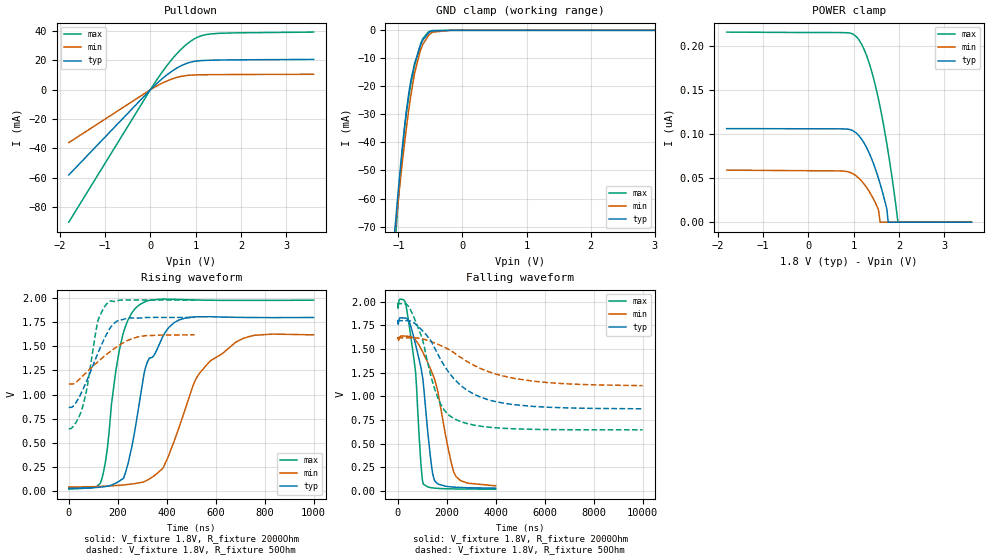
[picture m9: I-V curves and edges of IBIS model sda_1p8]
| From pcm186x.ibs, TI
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|   sda_1p8 Model
[Model]   sda_1p8
Model_type   I/O_open_drain
Polarity   Non-Inverting
Vinl = 0.54
Vinh = 1.26
Vmeas = 0.9
Vref = 1.8
Cref = 400pF
Rref = 2000
|   typ   min   max
|   (nom PVT)   (fast PVT)   (slow PVT)
C_comp   9.904e-12   9.661e-12   1.003e-11
[Model spec]
|subparameter
Vinl   0.54   0.486   0.594
Vinh   1.26   1.134   1.386
| Where nom  PVT is Nominal Process, 1.8V, 27C
|   Fast PVT is Strong Process,  1.98V, -40C
|   Slow PVT is Weak Process,   1.62V, 125C
[Voltage Range]   1.8   1.62   1.98
|Junction Temperature
[Temperature Range]   27   125   -40
[Pullup Reference]   1.8   1.62   1.98
[Pulldown Reference]   0   0   0
[Power Clamp Reference]   1.8   1.62   1.98
[GND Clamp Reference]   0   0   0
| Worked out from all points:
|   slope of the pulldown table from 0 to 0.27 V, typ, clamps not added: 34.7 ohm
|   GND clamp passes 1 mA (typ) near -0.53 V on its own axis
|   falling waveform, V_fixture 1.8V, R_fixture 2000Ohm: 20-80 % time 502ns typ, 817ns min, 358ns max; typ from 1.8 V to 0.031 V
|   rising waveform, V_fixture 1.8V, R_fixture 2000Ohm: 20-80 % time 105ns typ, 156ns min, 61.8ns max; typ from 0.028 V to 1.8 V
|   falling waveform, V_fixture 1.8V, R_fixture 50Ohm: 20-80 % time 1.62us typ, 2.39us min, 912ns max; typ from 1.8 V to 0.87 V
|   rising waveform, V_fixture 1.8V, R_fixture 50Ohm: 20-80 % time 94.1ns typ, 145ns min, 53.8ns max; typ from 0.868 V to 1.8 V
[Pulldown]
|   Voltage   I(typ)   I(min)   I(max)
-1.8V     -58.2mA    -36.13mA   -90.43mA
130.5mV   3.944mA    2.382mA    6.262mA
277mV     7.97mA     4.736mA    12.81mA
482.6mV   12.8mA     7.39mA     21.04mA
644.4mV   15.83mA    8.868mA    26.59mA
821.2mV   18.2mA     9.793mA    31.57mA
1.054V    19.71mA    10.17mA    36.04mA
1.331V    20.16mA    10.29mA    38.09mA
1.978V    20.42mA    10.4mA     38.88mA
3.6V      20.7mA     10.55mA    39.35mA
[GND Clamp]
|   Voltage   I(typ)   I(min)   I(max)
-1.8V     -364.4mA   -298.1mA   -450.1mA
-1.051V   -70.48mA   -71.85mA   -76.76mA
-1.003V   -57.72mA   -61.01mA   -61.48mA
-964.4mV  -48.15mA   -52.71mA   -50.3mA
-903.1mV  -34.39mA   -40.29mA   -35.2mA
-875mV    -28.89mA   -35mA      -29.71mA
-806.4mV  -18.17mA   -23.43mA   -19.44mA
-747mV    -11.85mA   -15.4mA    -12.68mA
-655.6mV  -5.372mA   -7.194mA   -5.046mA
-522.9mV  -763.3uA   -1.643mA   -392.6uA
-180mV    -66.44nA   -963.5nA   -79.79nA
3.6V      0A         0A         0A
[POWER Clamp]
|   Voltage   I(typ)   I(min)   I(max)
-1.8V     106.1nA    59.03nA    215.6nA
748.3mV   105.8nA    58.08nA    215nA
1.01V     102.9nA    54.12nA    212.5nA
1.237V    89.12nA    42.81nA    195.1nA
1.385V    73.37nA    31.25nA    173.3nA
1.485V    59.61nA    21.38nA    153.8nA
1.55V     49.37nA    13.69nA    139nA
1.584V    43.58nA    0A         130.7nA
1.732V    14.91nA    0A         88.82nA
1.762V    0A         0A         79.37nA
1.978V    0A         0A         0A
3.6V      0A         0A         0A
[Ramp]
R_load = 2000
|   typ   min   max
dV/dt_r   1.0624/1.05238e-07   0.946622/1.54408e-07   1.1752/6.13734e-08
dV/dt_f   1.06137/5.00852e-07   0.938568/8.14302e-07   1.17553/3.57285e-07
[Falling Waveform]
V_fixture = 1.8V
V_fixture_min = 1.62V
V_fixture_max = 1.98V
R_fixture = 2000Ohm
|   Time   V(typ)   V(min)   V(max)
0s        1.8V       1.62V      1.98V
296.4ns   1.828V     1.638V     2.003V
526.5ns   1.747V     1.632V     1.645V
731.1ns   1.546V     1.595V     1.253V
940.3ns   1.315V     1.509V     314.7mV
1.049us   1.128V     1.454V     73.04mV
1.334us   364mV      1.294V     37.38mV
1.501us   112.6mV    1.185V     31.46mV
2.379us   40.53mV    153.8mV    22.71mV
4us       30.84mV    55.6mV     20.35mV
[Rising Waveform]
V_fixture = 1.8V
V_fixture_min = 1.62V
V_fixture_max = 1.98V
R_fixture = 2000Ohm
|   Time   V(typ)   V(min)   V(max)
0s        28.42mV    41.71mV    19.91mV
129ns     40.85mV    48.74mV    81.17mV
206.7ns   103.6mV    60.02mV    1.463V
242.3ns   287.5mV    68.64mV    1.776V
288.3ns   915.3mV    85.71mV    1.931V
320.5ns   1.334V     113mV      1.971V
448.6ns   1.772V     646.8mV    1.987V
533ns     1.806V     1.219V     1.98V
680.9ns   1.801V     1.541V     1.977V
999.8ns   1.799V     1.619V     1.979V
[Falling Waveform]
V_fixture = 1.8V
V_fixture_min = 1.62V
V_fixture_max = 1.98V
R_fixture = 50Ohm
|   Time   V(typ)   V(min)   V(max)
0s        1.8V       1.62V      1.98V
532ns     1.795V     1.62V      1.91V
986ns     1.702V     1.61V      1.626V
1.386us   1.573V     1.577V     1.187V
1.644us   1.443V     1.551V     981.5mV
1.929us   1.314V     1.518V     846.2mV
2.332us   1.177V     1.456V     761.2mV
3.123us   1.023V     1.327V     697.1mV
4.321us   929.1mV    1.215V     663.4mV
9.999us   869.5mV    1.114V     646.8mV
[Rising Waveform]
V_fixture = 1.8V
V_fixture_min = 1.62V
V_fixture_max = 1.98V
R_fixture = 50Ohm
|   Time   V(typ)   V(min)   V(max)
0s        867.7mV    1.11V      646.7mV
27ns      908.3mV    1.123V     701.4mV
53ns      1.027V     1.183V     843.6mV
75ns      1.153V     1.236V     1.078V
117ns     1.417V     1.335V     1.743V
137ns     1.535V     1.38V      1.87V
162ns     1.661V     1.432V     1.959V
201ns     1.767V     1.503V     1.975V
285ns     1.793V     1.599V     1.98V
514ns     1.8V       1.62V      1.98V
